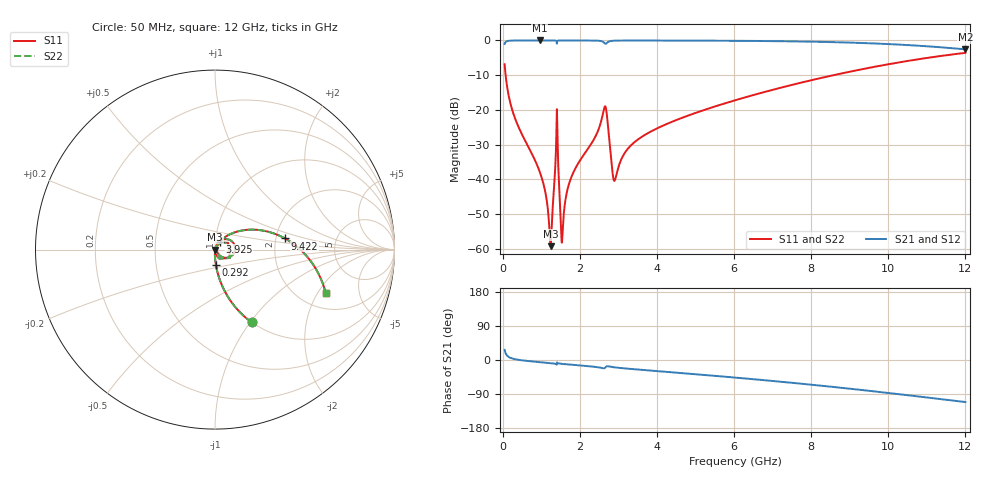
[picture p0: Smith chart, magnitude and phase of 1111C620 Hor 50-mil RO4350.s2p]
# GHz S MA R 50
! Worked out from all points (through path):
!   11951 points, 50 MHz to 12 GHz, reference 50 ohm
!   highest |S21| = -0.01 dB at 966 MHz (marker M1); lowest = -2.6 dB at 12 GHz (marker M2)
!   group delay of S21, straight-line fit = 25.9 ps
!   lowest |S11| = -59.3 dB at 1.242 GHz (marker M3), VSWR 1.00, Z = 50.1 - j0.0189 ohm
!   |S11| at or under -10 dB: 76.43 MHz to 8.586 GHz (8.509 GHz wide, 196 % of centre)
!   |S22| runs from -59.3 to -3.6 dB; largest |S21 - S12| = 0
!   S11 on the Smith chart (normalised r, x): 50 MHz: 0.99, -1.02; 292 MHz: 1.00, -0.17; 3.925 GHz: 1.05, +0.09; 9.422 GHz: 2.24, +0.33; 12 GHz: 2.74, -2.35
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0.05  0.4546 -63.3  0.8904 26.7  0.8904 26.7  0.4546 -63.3
0.292  0.08332 -86.8  0.996 2.8  0.996 2.8  0.08332 -86.8
0.966  0.01257 -91.9  0.999 -5.7  0.999 -5.7  0.01257 -91.9
1.242  0.001085 -10.0  0.9988 -8.3  0.9988 -8.3  0.001085 -10.0
1.285  0.002988 57.1  0.9987 -8.7  0.9987 -8.7  0.002988 57.1
1.36  0.01375 68.6  0.9971 -9.8  0.9971 -9.8  0.01375 68.6
1.393  0.04599 53.3  0.9795 -11.6  0.9795 -11.6  0.04599 53.3
1.435  0.0194 -84.1  0.9949 -8.5  0.9949 -8.5  0.0194 -84.1
1.497  0.003313 -75.0  0.9985 -9.8  0.9985 -9.8  0.003313 -75.0
1.547  0.001498 27.2  0.9987 -10.3  0.9987 -10.3  0.001498 27.2
1.719  0.008527 70.2  0.9987 -11.9  0.9987 -11.9  0.008527 70.2
2.042  0.02005 70.9  0.9981 -14.7  0.9981 -14.7  0.02005 70.9
2.642  0.1098 18.3  0.9129 -21.5  0.9129 -21.5  0.1098 18.3
2.903  0.009541 10.4  0.9915 -19.4  0.9915 -19.4  0.009541 10.4
3.247  0.02754 60.8  0.9964 -22.9  0.9964 -22.9  0.02754 60.8
3.925  0.05141 59.0  0.9963 -28.6  0.9963 -28.6  0.05141 59.0
4.034  0.05504 58.3  0.9961 -29.5  0.9961 -29.5  0.05504 58.3
6.025  0.1371 42.6  0.9877 -46.3  0.9877 -46.3  0.1371 42.6
8.017  0.2682 24.0  0.9597 -65.3  0.9597 -65.3  0.2682 24.0
9.422  0.3947 9.1  0.9144 -80.4  0.9144 -80.4  0.3947 9.1
10.009  0.4543 2.4  0.8861 -87.1  0.8861 -87.1  0.4543 2.4
12  0.6621 -21.4  0.7435 -110.9  0.7435 -110.9  0.6621 -21.4
